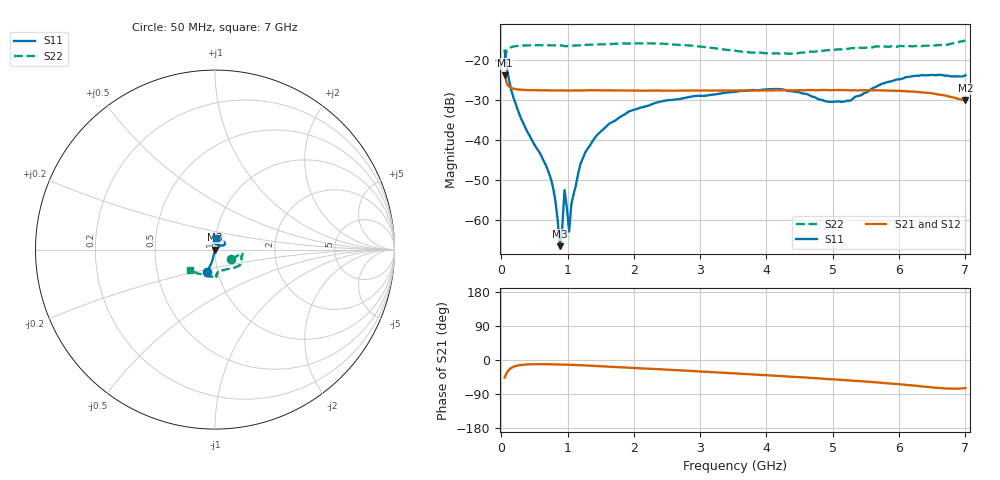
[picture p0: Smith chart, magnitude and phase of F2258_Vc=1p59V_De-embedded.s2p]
! Integrated Device Technology
! Corporate Headquarters
! 6024 Silver Creek Valley Road
! San Jose, CA 95138  USA
! Phone:  1-408-284-8200
! Toll Free:  1-800-223-1366
! Webpage:  http://www.idt.com/
! Timing and RF Division
! 515 Groton Road, Suite 102
! Westford, MA 01886-6024
! Device:  F2258
! Description: Voltage Variable RF Attenuator
! Frequency:  50.0 -  6000.00 MHz
! Package:  3x3 mm Thin QFN Plastic Package: 16 pin
! Ports:  2 RF, 2 DC
!  Pin  1  = NC
!  Pin  2  = NC
!  Pin  3  = RF2  = Port 2
!  Pin  4  = GND
!  Pin  5  = Vdd
!  Pin  6  = NC
!  Pin  7  = VCTRL
!  Pin  8  = NC
!  Pin  9  = GND
!  Pin 10  = RF1  = Port 1
!  Pin 11  = NC
!  Pin 12  = NC
!  Pin 13  = NC
!  Pin 14  = NC
!  Pin 15  = NC
!  Pin 16  = NC
! Vcntrl:  1.590 Volts
! Vdd:  +3.300 Volts
! Current:  1.159 mA
! Data:  The device was measured on a the F2258 evaluation board which has
!  individual transmission lines to the RF pins.  Data was collected
!  using a calibrated network analyzer.  The evaluation board was
!  de-embedded using a TRL calibration technique.
!  The reference plane is the edge of the package pin.
! Misc:  SN 10
!  Action Tracker AT0285
! Date Measured:  2014-12-10
! Date:  2016-01-13  MJV
! Note:
!  Integrated Device Technology supplies this data as a sample of measured
!  data at the package pin for this product.  Your particular data for this
!  product may vary.
!  Data was taken at 25 degrees C.
!  Integrated Device Technology reserves the right to change this data at anytime.
!Freq_(GHz)  S11M_(dB)  S11P_(deg)  S21M_(dB)  S21P_(deg)  S12M_(dB)  S12P_(deg)  S22M_(dB)  S22P_(deg)
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# GHz S dB R 50
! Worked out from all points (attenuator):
!   201 points, 50 MHz to 7 GHz, reference 50 ohm
!   highest |S21| = -23.67 dB at 50 MHz (marker M1); lowest = -30.0 dB at 7 GHz (marker M2)
!   lowest |S11| = -66.5 dB at 884 MHz (marker M3), VSWR 1.00, Z = 50 - j0.0178 ohm
!   |S11| at or under -10 dB: start of sweep to end of sweep
!   |S22| runs from -19.5 to -15.0 dB; largest |S21 - S12| = 0.00038
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0.05  -17.55 -109.3  -23.67 -46.2  -23.67 -46.2  -19.50 -30.5
0.1195  -25.17 -103.7  -26.59 -25.0  -26.59 -25.0  -16.88 -9.8
0.2585  -32.83 -104.5  -27.28 -14.2  -27.28 -14.2  -16.35 -7.0
0.745  -49.49 -101.6  -27.52 -11.3  -27.56 -11.3  -16.22 -11.7
0.8145  -55.01 -91.4  -27.52 -11.6  -27.55 -11.6  -16.23 -12.6
0.884  -66.47 -22.0  -27.50 -11.9  -27.54 -11.9  -16.25 -14.0
0.91875  -61.93 33.7  -27.50 -12.1  -27.54 -12.1  -16.26 -14.6
0.9535  -52.41 -119.5  -27.52 -12.3  -27.56 -12.3  -16.44 -14.3
1.023  -62.81 -55.7  -27.53 -12.6  -27.56 -12.6  -16.35 -15.7
1.05775  -55.81 -11.7  -27.51 -12.8  -27.56 -12.8  -16.32 -16.0
1.2315  -44.43 20.1  -27.51 -14.1  -27.55 -14.1  -16.15 -18.5
1.40525  -39.51 20.5  -27.46 -15.7  -27.53 -15.6  -16.04 -20.6
1.61375  -36.01 24.0  -27.48 -17.6  -27.53 -17.5  -15.90 -23.7
1.9265  -32.75 31.9  -27.53 -20.4  -27.58 -20.3  -15.76 -27.4
2.37825  -30.40 42.7  -27.58 -24.3  -27.58 -24.3  -15.78 -33.0
3.525  -27.87 89.1  -27.51 -35.4  -27.54 -35.3  -17.60 -54.5
4.1505  -27.14 103.9  -27.50 -41.7  -27.53 -41.7  -18.21 -72.4
4.7065  -29.11 94.2  -27.42 -47.6  -27.46 -47.5  -17.83 -83.0
5.2625  -30.09 50.5  -27.48 -53.9  -27.52 -53.8  -16.99 -86.6
5.85325  -25.33 27.4  -27.56 -61.9  -27.60 -61.9  -16.57 -88.4
6.33975  -23.65 33.2  -28.02 -69.7  -28.03 -69.7  -16.42 -98.7
7  -23.71 83.6  -29.99 -74.2  -30.05 -74.1  -15.00 -140.2
